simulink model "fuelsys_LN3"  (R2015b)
settings: Solver=ode45  SolverMode=SingleTasking  StartTime=0.0  StopTime=50  FixedStep=0.001  RelTol=1e-5  AbsTol=1e-6
PostLoadFcn:
  | sldemo_fuelsys_data(bdroot,'initialize_data','orig','float');
model workspace (MAT data in the model file):
  PressEst = [0.806253176324 0.553142316929 0.37151500209 0.277667903103 0.220198954207 0.181288665766 0.153200000489 0.115431020872 0.0913067476324 0.0746519188607 0.0625231108324 0.0533383634277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]
  PressVect = [0.05 0.1 0.15 0.2 0.25 0.3 0.35 0.4 0.45 0.5 0.55 0.6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]
  PumpCon = [-0.0556348 -0.0022828 0.0256932 0.0435188 0.0562692 0.0661194857143 0.0741572 0.08697 0.0972452 0.106070342857 0.1139892 0.121303866667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]
  RampRateKiX = [100 200 300 400 500 600]
  RampRateKiY = [0 0.2 0.4 0.6 0.8 1]
  RampRateKiZ = [0.012 0.024 0.036 0.048 0.06 0.072 0.024 0.048 0.072 0.096 0.12 0.144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]
  SpeedEst = [471.837839721 550.80940091 777.559313277 1080.9243499 1418.36795322 1769.7468768 2125.37309264 2480.20345067 2831.37796793 3177.14006959 3516.32917143 4064.90417867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]
  SpeedVect = [50 75 100 125 150 175 200 250 300 350 400 450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]
  ThrotEst = [0 0 0 0 0 0 0 0 0 0 0 0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]
  ThrotVect = [0 3 6 9 12 15 18 21 24 27 30 35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]
  hys = 25
  max_ego = 1.2
  max_press = 0.95
  max_speed = 628
  max_throt = 90
  min_press = 0.05
  min_speed = 50
  min_throt = 3
  st_range = 0.0001
  zero_thresh = 250
undefined symbols (not defined in the file or in its folder): DiscIntNeverNeededParam, sld_FuelModes, sldvsubsys
libraries: simulink x7, simulink_extras x2

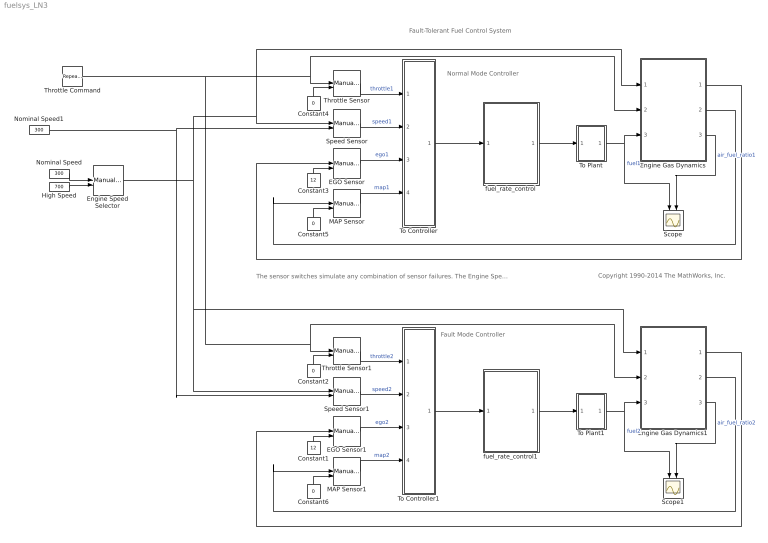
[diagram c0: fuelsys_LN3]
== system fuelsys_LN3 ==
  note: Normal Mode Controller
  note: Fault-Tolerant Fuel Control System
  note: Copyright 1990-2014 The MathWorks, Inc.
  note: The sensor switches simulate any combination of sensor failures. The Engine Speed Selector switch simulates different engine speeds (rad/sec).
  note: Fault Mode Controller
  Constant1 : Constant  Value=12
  Constant{2,4..6} (4 alike) : Constant  Value=0
  Constant3 : Constant  Value=12
  EGO Sensor : ManualSwitch
  EGO Sensor1 : ManualSwitch
  Engine Speed Selector : ManualSwitch
  Engine Gas Dynamics : Subsystem
  Engine Gas Dynamics1 : Subsystem
  High Speed : Constant  Value=700
  MAP Sensor : ManualSwitch
  MAP Sensor1 : ManualSwitch
  Nominal Speed : Constant  Value=300
  Nominal Speed1 : Constant  Value=300
  Scope : Scope  NumInputPorts=2
  Scope1 : Scope  NumInputPorts=2
  Speed Sensor : ManualSwitch  CurrentSetting=0
  Speed Sensor1 : ManualSwitch  CurrentSetting=0
  Throttle Command : simulink/Sources/Repeating Sequence  rep_seq_t=[0 2 4]  rep_seq_y=[10 20 10]
  Throttle Sensor : ManualSwitch
  Throttle Sensor1 : ManualSwitch
  To Controller : Subsystem
  To Controller1 : Subsystem
  To Plant : Subsystem
  To Plant1 : Subsystem
  fuel_rate_control : Subsystem  Tag=FuelRateControl  TreatAsAtomicUnit=on
  fuel_rate_control1 : Subsystem  Tag=FuelRateControl  TreatAsAtomicUnit=on
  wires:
  Engine Gas Dynamics/3(air/fuel ratio) -> Scope/2  "air_fuel_ratio1"
  fuel_rate_control/1(fuel_rate) -> To Plant/1(In1)
  Engine Gas Dynamics/1(o2_out) -> EGO Sensor/1
  Constant5/1 -> MAP Sensor/2
  Constant3/1 -> EGO Sensor/2
  Constant4/1 -> Throttle Sensor/2
  Engine Gas Dynamics/2(MAP) -> MAP Sensor/1
  High Speed/1 -> Engine Speed Selector/2
  Nominal Speed/1 -> Engine Speed Selector/1
  EGO Sensor/1 -> To Controller/3(ego)  "ego1"
  MAP Sensor/1 -> To Controller/4(map)  "map1"
  Throttle Sensor/1 -> To Controller/1(throttle)  "throttle1"
  Speed Sensor/1 -> To Controller/2(speed)  "speed1"
  To Plant/1(Out1) -> Scope/1, Engine Gas Dynamics/3(fuel)  "fuel1"
  To Controller/1(sensors) -> fuel_rate_control/1(sensors)
  Engine Gas Dynamics1/3(air/fuel ratio) -> Scope1/2  "air_fuel_ratio2"
  Engine Speed Selector/1 -> Engine Gas Dynamics/1(engine speed), Speed Sensor/1, Engine Gas Dynamics1/1(engine speed), Speed Sensor1/1
  fuel_rate_control1/1(fuel_rate) -> To Plant1/1(In1)
  Engine Gas Dynamics1/1(o2_out) -> EGO Sensor1/1
  Constant6/1 -> MAP Sensor1/2
  Constant1/1 -> EGO Sensor1/2
  Throttle Command/1 -> Engine Gas Dynamics/2(throttle angle), Throttle Sensor/1, Engine Gas Dynamics1/2(throttle angle), Throttle Sensor1/1
  Constant2/1 -> Throttle Sensor1/2
  Engine Gas Dynamics1/2(MAP) -> MAP Sensor1/1
  EGO Sensor1/1 -> To Controller1/3(ego)  "ego2"
  MAP Sensor1/1 -> To Controller1/4(map)  "map2"
  Throttle Sensor1/1 -> To Controller1/1(throttle)  "throttle2"
  Speed Sensor1/1 -> To Controller1/2(speed)  "speed2"
  To Plant1/1(Out1) -> Scope1/1, Engine Gas Dynamics1/3(fuel)  "fuel2"
  To Controller1/1(sensors) -> fuel_rate_control1/1(sensors)
  Nominal Speed1/1 -> Speed Sensor1/2, Speed Sensor/2

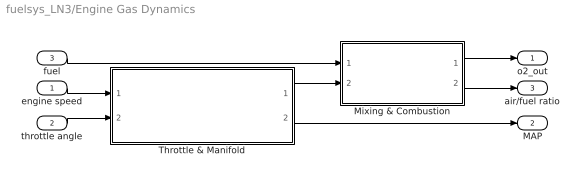
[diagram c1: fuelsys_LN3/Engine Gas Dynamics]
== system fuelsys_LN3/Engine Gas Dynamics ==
  engine speed : Inport
  throttle angle : Inport  Port=2
  fuel : Inport  Port=3
  Mixing & Combustion : Subsystem
  Throttle & Manifold : Subsystem
  o2_out : Outport
  MAP : Outport  Port=2
  air/fuel ratio : Outport  Port=3
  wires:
  Throttle & Manifold/1(Mass Airflow Rate) -> Mixing & Combustion/2(air flow)
  fuel/1 -> Mixing & Combustion/1(fuel rate)
  engine speed/1 -> Throttle & Manifold/1("Engine Speed, N")
  throttle angle/1 -> Throttle & Manifold/2(Throttle Ang.)
  Mixing & Combustion/2(air/fuel ratio) -> air/fuel ratio/1
  Throttle & Manifold/2(MAP (bar)) -> MAP/1
  Mixing & Combustion/1(o2_out) -> o2_out/1

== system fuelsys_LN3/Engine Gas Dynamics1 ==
  engine speed : Inport
  throttle angle : Inport  Port=2
  fuel : Inport  Port=3
  Mixing & Combustion : Subsystem
  Throttle & Manifold : Subsystem
  o2_out : Outport
  MAP : Outport  Port=2
  air/fuel ratio : Outport  Port=3
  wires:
  Throttle & Manifold/1(Mass Airflow Rate) -> Mixing & Combustion/2(air flow)
  fuel/1 -> Mixing & Combustion/1(fuel rate)
  engine speed/1 -> Throttle & Manifold/1("Engine Speed, N")
  throttle angle/1 -> Throttle & Manifold/2(Throttle Ang.)
  Mixing & Combustion/2(air/fuel ratio) -> air/fuel ratio/1
  Throttle & Manifold/2(MAP (bar)) -> MAP/1
  Mixing & Combustion/1(o2_out) -> o2_out/1

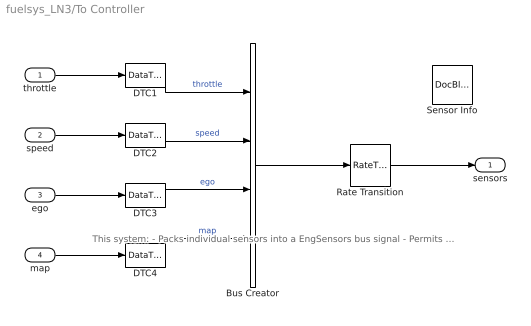
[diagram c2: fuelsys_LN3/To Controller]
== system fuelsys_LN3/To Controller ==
  note: This system: - Packs individual sensors into a EngSensors bus signal - Permits bus elements data types to change - Converts signals from continuous to discrete time
  throttle : Inport
  speed : Inport  Port=2
  ego : Inport  Port=3
  map : Inport  Port=4
  Bus Creator : BusCreator  Inputs=4  OutDataTypeStr=Bus: EngSensors
  DTC{1..4} (4 alike) : DataTypeConversion  SampleTime=[0 1]
  Rate Transition : RateTransition  OutPortSampleTime=0.01
  Sensor Info : simulink/Model-Wide Utilities/DocBlock  DocumentType=Text
  sensors : Outport
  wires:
  throttle/1 -> DTC1/1
  DTC1/1 -> Bus Creator/1  "throttle"
  speed/1 -> DTC2/1
  DTC2/1 -> Bus Creator/2  "speed"
  ego/1 -> DTC3/1
  DTC3/1 -> Bus Creator/3  "ego"
  map/1 -> DTC4/1
  DTC4/1 -> Bus Creator/4  "map"
  Bus Creator/1 -> Rate Transition/1
  Rate Transition/1 -> sensors/1

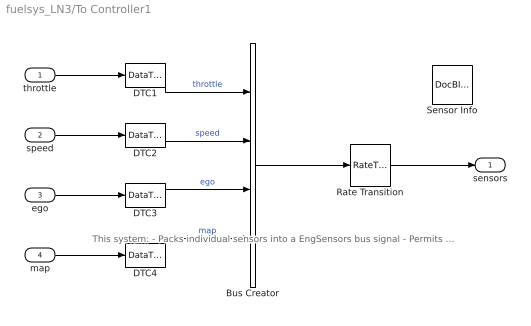
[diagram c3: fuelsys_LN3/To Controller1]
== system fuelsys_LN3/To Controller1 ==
  note: This system: - Packs individual sensors into a EngSensors bus signal - Permits bus elements data types to change - Converts signals from continuous to discrete time
  throttle : Inport
  speed : Inport  Port=2
  ego : Inport  Port=3
  map : Inport  Port=4
  Bus Creator : BusCreator  Inputs=4  OutDataTypeStr=Bus: EngSensors
  DTC{1..4} (4 alike) : DataTypeConversion  SampleTime=[0 1]
  Rate Transition : RateTransition  OutPortSampleTime=0.01
  Sensor Info : simulink/Model-Wide Utilities/DocBlock  DocumentType=Text
  sensors : Outport
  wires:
  throttle/1 -> DTC1/1
  DTC1/1 -> Bus Creator/1  "throttle"
  speed/1 -> DTC2/1
  DTC2/1 -> Bus Creator/2  "speed"
  ego/1 -> DTC3/1
  DTC3/1 -> Bus Creator/3  "ego"
  map/1 -> DTC4/1
  DTC4/1 -> Bus Creator/4  "map"
  Bus Creator/1 -> Rate Transition/1
  Rate Transition/1 -> sensors/1

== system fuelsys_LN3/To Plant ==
  note: This system: - Permits upstream signal data type to change - Converts signals from discrete to continuous time
  In1 : Inport
  DTC5 : DataTypeConversion
  Rate Transition1 : RateTransition  Integrity=off  X0=1.6  OutPortSampleTime=0
  Out1 : Outport
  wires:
  DTC5/1 -> Rate Transition1/1
  In1/1 -> DTC5/1
  Rate Transition1/1 -> Out1/1

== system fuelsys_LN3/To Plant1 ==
  note: This system: - Permits upstream signal data type to change - Converts signals from discrete to continuous time
  In1 : Inport
  DTC5 : DataTypeConversion
  Rate Transition1 : RateTransition  Integrity=off  X0=1.6  OutPortSampleTime=0
  Out1 : Outport
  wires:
  DTC5/1 -> Rate Transition1/1
  In1/1 -> DTC5/1
  Rate Transition1/1 -> Out1/1

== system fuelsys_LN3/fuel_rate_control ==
  note: Fuel Rate Control Subsystem
  sensors : Inport  OutDataTypeStr=Bus: EngSensors
  Bus Selector1 : BusSelector  OutputSignals=speed
  airflow_calc : Subsystem
  control_logic : Stateflow chart  Description=Stateflow diagram to determine control system operating mode  TreatAsAtomicUnit=on
  fuel_calc : Subsystem
  validate_sample_time : Subsystem  Tag=VerificationSubsystem  DisableCoverage=on  LoadFcn=sldvsubsys('check')  TreatAsAtomicUnit=on  SimViewingDevice=on
  fuel_rate : Outport
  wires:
  fuel_calc/1(fuel_rate) -> fuel_rate/1
  airflow_calc/1(est_airflow) -> fuel_calc/1(est_airflow)
  sensors/1 -> control_logic/1(es_i), Bus Selector1/1
  control_logic/3(fuel_mode) -> airflow_calc/3(fuel_mode), fuel_calc/3(fuel_mode)
  control_logic/1(es_o) -> airflow_calc/1(sensors)
  control_logic/2(" O2_normal") -> airflow_calc/2(O2_normal)
  airflow_calc/2(fb_correction) -> fuel_calc/2(fb_correction)
  Bus Selector1/1 -> validate_sample_time/1(In1)  "<speed>"

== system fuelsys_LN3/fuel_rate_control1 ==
  note: Fuel Rate Control Subsystem
  sensors : Inport  OutDataTypeStr=Bus: EngSensors
  Bus Selector1 : BusSelector  OutputSignals=speed
  airflow_calc : Subsystem
  control_logic : Stateflow chart  Description=Stateflow diagram to determine control system operating mode  TreatAsAtomicUnit=on
  fuel_calc : Subsystem
  validate_sample_time : Subsystem  Tag=VerificationSubsystem  DisableCoverage=on  LoadFcn=sldvsubsys('check')  TreatAsAtomicUnit=on  SimViewingDevice=on
  fuel_rate : Outport
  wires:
  fuel_calc/1(fuel_rate) -> fuel_rate/1
  airflow_calc/1(est_airflow) -> fuel_calc/1(est_airflow)
  sensors/1 -> control_logic/1(es_i), Bus Selector1/1
  control_logic/3(fuel_mode) -> airflow_calc/3(fuel_mode), fuel_calc/3(fuel_mode)
  control_logic/1(es_o) -> airflow_calc/1(sensors)
  control_logic/2(" O2_normal") -> airflow_calc/2(O2_normal)
  airflow_calc/2(fb_correction) -> fuel_calc/2(fb_correction)
  Bus Selector1/1 -> validate_sample_time/1(In1)  "<speed>"

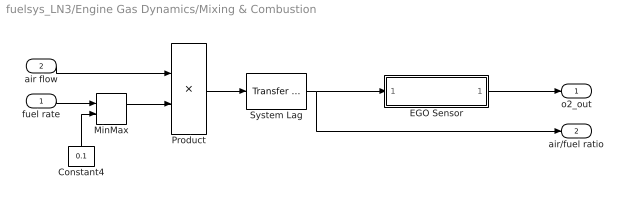
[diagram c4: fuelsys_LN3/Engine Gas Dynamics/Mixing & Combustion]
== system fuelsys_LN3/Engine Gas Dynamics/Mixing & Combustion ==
  fuel rate : Inport
  air flow : Inport  Port=2
  Constant4 : Constant  Value=0.1
  EGO Sensor : MATLAB Function  TreatAsAtomicUnit=on
  MinMax : MinMax  Function=max  Inputs=2
  Product : Product  Inputs=*/
  System Lag : simulink_extras/Additional Linear/Transfer Fcn (with initial outputs)  N=3  D=[1 3]  Y0=1/14.6  U0=1/14.6
  o2_out : Outport
  air/fuel ratio : Outport  Port=2
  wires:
  Constant4/1 -> MinMax/2
  fuel rate/1 -> MinMax/1
  MinMax/1 -> Product/2
  Product/1 -> System Lag/1
  System Lag/1 -> air/fuel ratio/1, EGO Sensor/1(u)
  EGO Sensor/1(y) -> o2_out/1
  air flow/1 -> Product/1

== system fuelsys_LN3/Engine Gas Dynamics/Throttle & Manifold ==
  note: Air-Fuel Intake Dynamics
  "Engine Speed, N" : Inport
  Throttle Ang. : Inport  Port=2
  "Atmospheric Pressure, Pa (bar)" : Constant  Value=1.0
  Intake Manifold : Subsystem
  Limit to Positive : Saturate  UpperLimit=inf  LowerLimit=0
  Throttle : Subsystem
  Mass Airflow Rate : Outport
  MAP (bar) : Outport  Port=2
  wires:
  Limit to Positive/1 -> Throttle/1("Throttle Angle, theta (deg)")
  Throttle Ang./1 -> Limit to Positive/1
  Throttle/1("Throttle Flow, mdot (g/s)") -> Intake Manifold/1(mdot Input (g/s))
  "Engine Speed, N"/1 -> Intake Manifold/2(N (rad/sec))
  Intake Manifold/1(mdot to Cylinder (g/s)) -> Mass Airflow Rate/1
  "Atmospheric Pressure, Pa (bar)"/1 -> Throttle/3("Atmospheric Pressure, Pa (bar) ")
  Intake Manifold/2("Manifold Pressure, Pm (bar)") -> Throttle/2("Manifold Pressure, Pm (bar)"), MAP (bar)/1

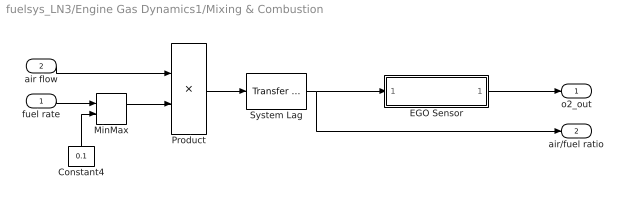
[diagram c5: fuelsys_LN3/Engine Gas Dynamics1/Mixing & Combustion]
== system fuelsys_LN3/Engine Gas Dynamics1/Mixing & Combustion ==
  fuel rate : Inport
  air flow : Inport  Port=2
  Constant4 : Constant  Value=0.1
  EGO Sensor : MATLAB Function  TreatAsAtomicUnit=on
  MinMax : MinMax  Function=max  Inputs=2
  Product : Product  Inputs=*/
  System Lag : simulink_extras/Additional Linear/Transfer Fcn (with initial outputs)  N=3  D=[1 3]  Y0=1/14.6  U0=1/14.6
  o2_out : Outport
  air/fuel ratio : Outport  Port=2
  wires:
  Constant4/1 -> MinMax/2
  fuel rate/1 -> MinMax/1
  MinMax/1 -> Product/2
  Product/1 -> System Lag/1
  System Lag/1 -> air/fuel ratio/1, EGO Sensor/1(u)
  EGO Sensor/1(y) -> o2_out/1
  air flow/1 -> Product/1

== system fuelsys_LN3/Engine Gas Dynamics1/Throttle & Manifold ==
  note: Air-Fuel Intake Dynamics
  "Engine Speed, N" : Inport
  Throttle Ang. : Inport  Port=2
  "Atmospheric Pressure, Pa (bar)" : Constant  Value=1.0
  Intake Manifold : Subsystem
  Limit to Positive : Saturate  UpperLimit=inf  LowerLimit=0
  Throttle : Subsystem
  Mass Airflow Rate : Outport
  MAP (bar) : Outport  Port=2
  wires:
  Limit to Positive/1 -> Throttle/1("Throttle Angle, theta (deg)")
  Throttle Ang./1 -> Limit to Positive/1
  Throttle/1("Throttle Flow, mdot (g/s)") -> Intake Manifold/1(mdot Input (g/s))
  "Engine Speed, N"/1 -> Intake Manifold/2(N (rad/sec))
  Intake Manifold/1(mdot to Cylinder (g/s)) -> Mass Airflow Rate/1
  "Atmospheric Pressure, Pa (bar)"/1 -> Throttle/3("Atmospheric Pressure, Pa (bar) ")
  Intake Manifold/2("Manifold Pressure, Pm (bar)") -> Throttle/2("Manifold Pressure, Pm (bar)"), MAP (bar)/1

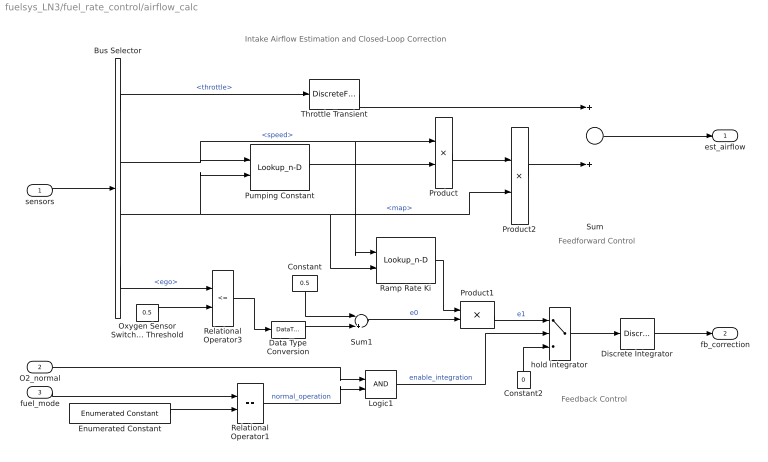
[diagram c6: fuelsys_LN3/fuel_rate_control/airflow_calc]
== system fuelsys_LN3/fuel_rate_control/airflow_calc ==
  note: Intake Airflow Estimation and Closed-Loop Correction
  note: Feedback Control
  note: Feedforward Control
  sensors : Inport
  O2_normal : Inport  Port=2
  fuel_mode : Inport  Port=3
  Bus Selector : BusSelector  OutputSignals=throttle,speed,map,ego
  Constant : Constant  Value=0.5  OutDataTypeStr=s16En7
  Constant2 : Constant  Value=0  OutDataTypeStr=uint8
  Data Type Conversion : DataTypeConversion  OutDataTypeStr=s16En7  RndMeth=Simplest
  Discrete Integrator : DiscreteIntegrator  InitialConditionSetting=State (most efficient)  SampleTime=-1  OutDataTypeStr=s16En15  RndMeth=Simplest  ICPrevOutput=DiscIntNeverNeededParam  ICPrevScaledInput=DiscIntNeverNeededParam
  Enumerated Constant : simulink/Sources/Enumerated Constant  OutDataTypeStr=Enum: sld_FuelModes  Value=sld_FuelModes.LOW  SampleTime=.01
  Logic1 : Logic  IconShape=distinctive  AllPortsSameDT=off  OutDataTypeStr=boolean
  Oxygen Sensor Switching Threshold : Constant  Value=0.5  OutDataTypeStr=s16En7
  Product : Product  OutDataTypeStr=s16En7  RndMeth=Simplest
  Product1 : Product  OutDataTypeStr=s16En15  RndMeth=Simplest
  Product2 : Product  OutDataTypeStr=s16En7  RndMeth=Simplest
  Pumping Constant : Lookup_n-D  BreakpointsForDimension1=SpeedVect  BreakpointsForDimension2=PressVect  IndexSearchMethod=Linear search  Table=PumpCon  ExtrapMethod=Clip  UseLastTableValue=on  OutDataTypeStr=s16En15  RndMeth=Simplest
  Ramp Rate Ki : Lookup_n-D  BreakpointsForDimension1=RampRateKiX  BreakpointsForDimension2=RampRateKiY  IndexSearchMethod=Linear search  Table=RampRateKiZ  ExtrapMethod=Clip  UseLastTableValue=on  OutDataTypeStr=s16En15  RndMeth=Simplest
  Relational Operator1 : RelationalOperator  Operator===  OutDataTypeStr=boolean
  Relational Operator3 : RelationalOperator  Operator=<=  OutDataTypeStr=boolean
  Sum : Sum  Inputs=2  OutDataTypeStr=s16En7  RndMeth=Simplest
  Sum1 : Sum  Inputs=-+  OutDataTypeStr=s16En15  RndMeth=Simplest
  Throttle Transient : DiscreteFilter  Numerator=[.01 -.01]  Denominator=[1 -.8]  a0EqualsOne=on  OutDataTypeStr=s16En7  RndMeth=Simplest
  hold integrator : Switch  Criteria=u2 ~= 0  Threshold=1  OutDataTypeStr=s16En15  RndMeth=Simplest
  est_airflow : Outport
  fb_correction : Outport  Port=2
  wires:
  Discrete Integrator/1 -> fb_correction/1
  sensors/1 -> Bus Selector/1
  Pumping Constant/1 -> Product/2
  Bus Selector/2 -> Product/1, Ramp Rate Ki/1, Pumping Constant/1  "<speed>"
  Throttle Transient/1 -> Sum/1
  Sum/1 -> est_airflow/1
  Bus Selector/1 -> Throttle Transient/1  "<throttle>"
  Relational Operator1/1 -> Logic1/2  "normal_operation"
  Oxygen Sensor Switching Threshold/1 -> Relational Operator3/2
  Constant/1 -> Sum1/1
  Ramp Rate Ki/1 -> Product1/1
  Constant2/1 -> hold integrator/3
  Product1/1 -> hold integrator/1  "e1"
  hold integrator/1 -> Discrete Integrator/1
  Logic1/1 -> hold integrator/2  "enable_integration"
  Sum1/1 -> Product1/2  "e0"
  Relational Operator3/1 -> Data Type Conversion/1
  Data Type Conversion/1 -> Sum1/2
  Bus Selector/3 -> Product2/2, Ramp Rate Ki/2, Pumping Constant/2  "<map>"
  Bus Selector/4 -> Relational Operator3/1  "<ego>"
  Product/1 -> Product2/1
  Product2/1 -> Sum/2
  O2_normal/1 -> Logic1/1
  Enumerated Constant/1 -> Relational Operator1/2
  fuel_mode/1 -> Relational Operator1/1

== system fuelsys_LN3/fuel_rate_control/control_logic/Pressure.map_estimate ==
  note: MAP Estimation
  speed : Inport  OutDataTypeStr=s16En3
  throttle : Inport  Port=2  OutDataTypeStr=s16En3
  f : TriggerPort  TriggerType=function-call
  Pressure Estimation : Lookup_n-D  BreakpointsForDimension1=SpeedVect  BreakpointsForDimension2=ThrotVect  IndexSearchMethod=Linear search  Table=PressEst  ExtrapMethod=Clip  UseLastTableValue=on  OutDataTypeStr=u8En7  RndMeth=Simplest
  map : Outport
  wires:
  speed/1 -> Pressure Estimation/1
  throttle/1 -> Pressure Estimation/2
  Pressure Estimation/1 -> map/1

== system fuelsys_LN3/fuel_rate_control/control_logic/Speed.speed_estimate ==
  note: Speed Estimation
  throttle : Inport  OutDataTypeStr=s16En3
  map : Inport  Port=2  OutDataTypeStr=u8En7
  f : TriggerPort  TriggerType=function-call
  Saturation : Saturate  UpperLimit=max_speed  LowerLimit=0  OutDataTypeStr=s16En3
  Speed Estimation : Lookup_n-D  BreakpointsForDimension1=ThrotVect  BreakpointsForDimension2=PressVect  IndexSearchMethod=Linear search  Table=SpeedEst  ExtrapMethod=Clip  UseLastTableValue=on  OutDataTypeStr=s16En3  RndMeth=Simplest
  speed : Outport
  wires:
  Speed Estimation/1 -> Saturation/1
  throttle/1 -> Speed Estimation/1
  map/1 -> Speed Estimation/2
  Saturation/1 -> speed/1

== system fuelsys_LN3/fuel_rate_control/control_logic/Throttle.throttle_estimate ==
  note: Throttle Estimation
  speed : Inport  OutDataTypeStr=s16En3
  map : Inport  Port=2  OutDataTypeStr=u8En7
  f : TriggerPort  TriggerType=function-call
  Throttle Estimation : Lookup_n-D  BreakpointsForDimension1=SpeedVect  BreakpointsForDimension2=PressVect  IndexSearchMethod=Linear search  Table=ThrotEst  ExtrapMethod=Clip  UseLastTableValue=on  OutDataTypeStr=s16En7  RndMeth=Simplest
  throttle : Outport
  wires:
  speed/1 -> Throttle Estimation/1
  map/1 -> Throttle Estimation/2
  Throttle Estimation/1 -> throttle/1

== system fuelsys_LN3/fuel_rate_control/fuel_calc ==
  note: Fuel Rate Calculation
  est_airflow : Inport
  fb_correction : Inport  Port=2
  fuel_mode : Inport  Port=3
  feedforward_fuel_rate : Subsystem
  switchable_compensation : Subsystem
  fuel_rate : Outport
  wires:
  est_airflow/1 -> feedforward_fuel_rate/1(est_airflow)
  fuel_mode/1 -> feedforward_fuel_rate/2(fuel_mode), switchable_compensation/2(fuel_mode)
  switchable_compensation/1(fuel_rate) -> fuel_rate/1
  fb_correction/1 -> switchable_compensation/3(fb_correction)
  feedforward_fuel_rate/1(ff_fuel_rate) -> switchable_compensation/1(ff_fuel_rate)

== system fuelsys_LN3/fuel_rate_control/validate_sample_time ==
  note: The contents of this subsystem are excluded from the code Simulink Coder generates. To work correctly this system must continue to * Contain no output ports * Enable its 'Treat as Atomic Unit' parameter * Specify its 'Mask type' parameter as "VerificationSubsystem"
  note: Verify sample time: aspects of the design assume a 0.01 second sample time.
  In1 : Inport
  Actual Sample Time : Probe  ProbeWidth=off  ProbeComplexSignal=off  ProbeSampleTimeDataType=Same as input
  CheckRange : simulink/Model Verification/Check  Static Range  Description=-st_range < u < st_range  max=st_range  max_included=off  min=-st_range  min_included=off  enabled=on  stopWhenAssertionFail=on  export=off  icon=graphic
  Data Type Conversion : DataTypeConversion  OutDataTypeStr=s16En15
  Demux : Demux  Outputs=2
  Expected Sample Time : Constant  Value=0.01  OutDataTypeStr=s16En15
  Sum : Sum  Inputs=|+-
  Terminator : Terminator
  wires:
  Actual Sample Time/1 -> Demux/1
  In1/1 -> Data Type Conversion/1
  Demux/2 -> Terminator/1
  Demux/1 -> Sum/1
  Expected Sample Time/1 -> Sum/2
  Sum/1 -> CheckRange/1
  Data Type Conversion/1 -> Actual Sample Time/1

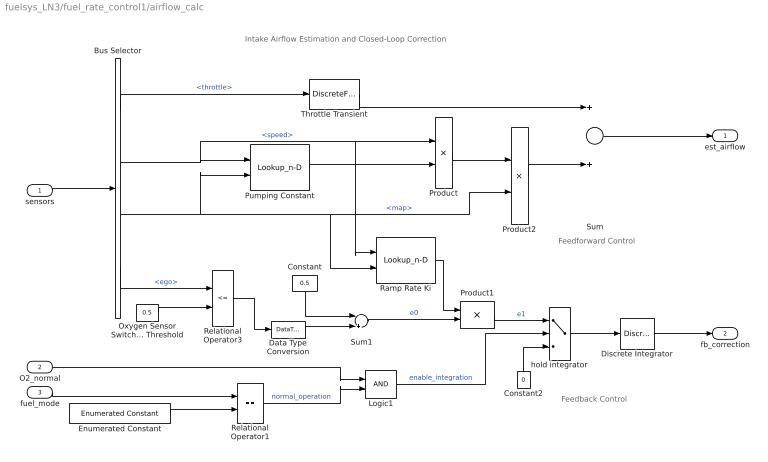
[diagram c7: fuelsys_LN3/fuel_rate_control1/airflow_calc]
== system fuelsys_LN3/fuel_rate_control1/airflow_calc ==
  note: Intake Airflow Estimation and Closed-Loop Correction
  note: Feedback Control
  note: Feedforward Control
  sensors : Inport
  O2_normal : Inport  Port=2
  fuel_mode : Inport  Port=3
  Bus Selector : BusSelector  OutputSignals=throttle,speed,map,ego
  Constant : Constant  Value=0.5  OutDataTypeStr=s16En7
  Constant2 : Constant  Value=0  OutDataTypeStr=uint8
  Data Type Conversion : DataTypeConversion  OutDataTypeStr=s16En7  RndMeth=Simplest
  Discrete Integrator : DiscreteIntegrator  InitialConditionSetting=State (most efficient)  SampleTime=-1  OutDataTypeStr=s16En15  RndMeth=Simplest  ICPrevOutput=DiscIntNeverNeededParam  ICPrevScaledInput=DiscIntNeverNeededParam
  Enumerated Constant : simulink/Sources/Enumerated Constant  OutDataTypeStr=Enum: sld_FuelModes  Value=sld_FuelModes.LOW  SampleTime=.01
  Logic1 : Logic  IconShape=distinctive  AllPortsSameDT=off  OutDataTypeStr=boolean
  Oxygen Sensor Switching Threshold : Constant  Value=0.5  OutDataTypeStr=s16En7
  Product : Product  OutDataTypeStr=s16En7  RndMeth=Simplest
  Product1 : Product  OutDataTypeStr=s16En15  RndMeth=Simplest
  Product2 : Product  OutDataTypeStr=s16En7  RndMeth=Simplest
  Pumping Constant : Lookup_n-D  BreakpointsForDimension1=SpeedVect  BreakpointsForDimension2=PressVect  IndexSearchMethod=Linear search  Table=PumpCon  ExtrapMethod=Clip  UseLastTableValue=on  OutDataTypeStr=s16En15  RndMeth=Simplest
  Ramp Rate Ki : Lookup_n-D  BreakpointsForDimension1=RampRateKiX  BreakpointsForDimension2=RampRateKiY  IndexSearchMethod=Linear search  Table=RampRateKiZ  ExtrapMethod=Clip  UseLastTableValue=on  OutDataTypeStr=s16En15  RndMeth=Simplest
  Relational Operator1 : RelationalOperator  Operator===  OutDataTypeStr=boolean
  Relational Operator3 : RelationalOperator  Operator=<=  OutDataTypeStr=boolean
  Sum : Sum  Inputs=2  OutDataTypeStr=s16En7  RndMeth=Simplest
  Sum1 : Sum  Inputs=-+  OutDataTypeStr=s16En15  RndMeth=Simplest
  Throttle Transient : DiscreteFilter  Numerator=[.01 -.01]  Denominator=[1 -.8]  a0EqualsOne=on  OutDataTypeStr=s16En7  RndMeth=Simplest
  hold integrator : Switch  Criteria=u2 ~= 0  Threshold=1  OutDataTypeStr=s16En15  RndMeth=Simplest
  est_airflow : Outport
  fb_correction : Outport  Port=2
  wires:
  Discrete Integrator/1 -> fb_correction/1
  sensors/1 -> Bus Selector/1
  Pumping Constant/1 -> Product/2
  Bus Selector/2 -> Product/1, Ramp Rate Ki/1, Pumping Constant/1  "<speed>"
  Throttle Transient/1 -> Sum/1
  Sum/1 -> est_airflow/1
  Bus Selector/1 -> Throttle Transient/1  "<throttle>"
  Relational Operator1/1 -> Logic1/2  "normal_operation"
  Oxygen Sensor Switching Threshold/1 -> Relational Operator3/2
  Constant/1 -> Sum1/1
  Ramp Rate Ki/1 -> Product1/1
  Constant2/1 -> hold integrator/3
  Product1/1 -> hold integrator/1  "e1"
  hold integrator/1 -> Discrete Integrator/1
  Logic1/1 -> hold integrator/2  "enable_integration"
  Sum1/1 -> Product1/2  "e0"
  Relational Operator3/1 -> Data Type Conversion/1
  Data Type Conversion/1 -> Sum1/2
  Bus Selector/3 -> Product2/2, Ramp Rate Ki/2, Pumping Constant/2  "<map>"
  Bus Selector/4 -> Relational Operator3/1  "<ego>"
  Product/1 -> Product2/1
  Product2/1 -> Sum/2
  O2_normal/1 -> Logic1/1
  Enumerated Constant/1 -> Relational Operator1/2
  fuel_mode/1 -> Relational Operator1/1

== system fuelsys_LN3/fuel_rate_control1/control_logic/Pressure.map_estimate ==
  note: MAP Estimation
  speed : Inport  OutDataTypeStr=s16En3
  throttle : Inport  Port=2  OutDataTypeStr=s16En3
  f : TriggerPort  TriggerType=function-call
  Pressure Estimation : Lookup_n-D  BreakpointsForDimension1=SpeedVect  BreakpointsForDimension2=ThrotVect  IndexSearchMethod=Linear search  Table=PressEst  ExtrapMethod=Clip  UseLastTableValue=on  OutDataTypeStr=u8En7  RndMeth=Simplest
  map : Outport
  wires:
  speed/1 -> Pressure Estimation/1
  throttle/1 -> Pressure Estimation/2
  Pressure Estimation/1 -> map/1

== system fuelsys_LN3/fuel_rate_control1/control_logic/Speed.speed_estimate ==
  note: Speed Estimation
  throttle : Inport  OutDataTypeStr=s16En3
  map : Inport  Port=2  OutDataTypeStr=u8En7
  f : TriggerPort  TriggerType=function-call
  Saturation : Saturate  UpperLimit=max_speed  LowerLimit=0  OutDataTypeStr=s16En3
  Speed Estimation : Lookup_n-D  BreakpointsForDimension1=ThrotVect  BreakpointsForDimension2=PressVect  IndexSearchMethod=Linear search  Table=SpeedEst  ExtrapMethod=Clip  UseLastTableValue=on  OutDataTypeStr=s16En3  RndMeth=Simplest
  speed : Outport
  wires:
  Speed Estimation/1 -> Saturation/1
  throttle/1 -> Speed Estimation/1
  map/1 -> Speed Estimation/2
  Saturation/1 -> speed/1

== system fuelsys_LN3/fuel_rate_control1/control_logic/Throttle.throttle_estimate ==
  note: Throttle Estimation
  speed : Inport  OutDataTypeStr=s16En3
  map : Inport  Port=2  OutDataTypeStr=u8En7
  f : TriggerPort  TriggerType=function-call
  Throttle Estimation : Lookup_n-D  BreakpointsForDimension1=SpeedVect  BreakpointsForDimension2=PressVect  IndexSearchMethod=Linear search  Table=ThrotEst  ExtrapMethod=Clip  UseLastTableValue=on  OutDataTypeStr=s16En7  RndMeth=Simplest
  throttle : Outport
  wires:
  speed/1 -> Throttle Estimation/1
  map/1 -> Throttle Estimation/2
  Throttle Estimation/1 -> throttle/1

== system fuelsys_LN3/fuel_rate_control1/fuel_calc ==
  note: Fuel Rate Calculation
  est_airflow : Inport
  fb_correction : Inport  Port=2
  fuel_mode : Inport  Port=3
  feedforward_fuel_rate : Subsystem
  switchable_compensation : Subsystem
  fuel_rate : Outport
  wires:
  est_airflow/1 -> feedforward_fuel_rate/1(est_airflow)
  fuel_mode/1 -> feedforward_fuel_rate/2(fuel_mode), switchable_compensation/2(fuel_mode)
  switchable_compensation/1(fuel_rate) -> fuel_rate/1
  fb_correction/1 -> switchable_compensation/3(fb_correction)
  feedforward_fuel_rate/1(ff_fuel_rate) -> switchable_compensation/1(ff_fuel_rate)

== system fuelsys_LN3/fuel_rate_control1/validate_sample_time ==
  note: The contents of this subsystem are excluded from the code Simulink Coder generates. To work correctly this system must continue to * Contain no output ports * Enable its 'Treat as Atomic Unit' parameter * Specify its 'Mask type' parameter as "VerificationSubsystem"
  note: Verify sample time: aspects of the design assume a 0.01 second sample time.
  In1 : Inport
  Actual Sample Time : Probe  ProbeWidth=off  ProbeComplexSignal=off  ProbeSampleTimeDataType=Same as input
  CheckRange : simulink/Model Verification/Check  Static Range  Description=-st_range < u < st_range  max=st_range  max_included=off  min=-st_range  min_included=off  enabled=on  stopWhenAssertionFail=on  export=off  icon=graphic
  Data Type Conversion : DataTypeConversion  OutDataTypeStr=s16En15
  Demux : Demux  Outputs=2
  Expected Sample Time : Constant  Value=0.01  OutDataTypeStr=s16En15
  Sum : Sum  Inputs=|+-
  Terminator : Terminator
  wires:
  Actual Sample Time/1 -> Demux/1
  In1/1 -> Data Type Conversion/1
  Demux/2 -> Terminator/1
  Demux/1 -> Sum/1
  Expected Sample Time/1 -> Sum/2
  Sum/1 -> CheckRange/1
  Data Type Conversion/1 -> Actual Sample Time/1

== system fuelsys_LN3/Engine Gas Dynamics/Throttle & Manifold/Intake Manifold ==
  note: Intake Manifold Vacuum
  mdot Input (g/s) : Inport
  N (rad/sec) : Inport  Port=2
  MATLAB Function : MATLAB Function  TreatAsAtomicUnit=on
  RT/Vm : Gain  Gain=0.41328
  Sum : Sum  Inputs=+-
  p0 = 0.589 bar : Integrator  InitialCondition=.589
  mdot to Cylinder (g/s) : Outport
  "Manifold Pressure, Pm (bar)" : Outport  Port=2
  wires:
  mdot Input (g/s)/1 -> Sum/1
  RT/Vm/1 -> p0 = 0.589 bar/1
  N (rad/sec)/1 -> MATLAB Function/2(u2)
  p0 = 0.589 bar/1 -> "Manifold Pressure, Pm (bar)"/1, MATLAB Function/1(u1)
  Sum/1 -> RT/Vm/1
  MATLAB Function/1(y) -> mdot to Cylinder (g/s)/1, Sum/2

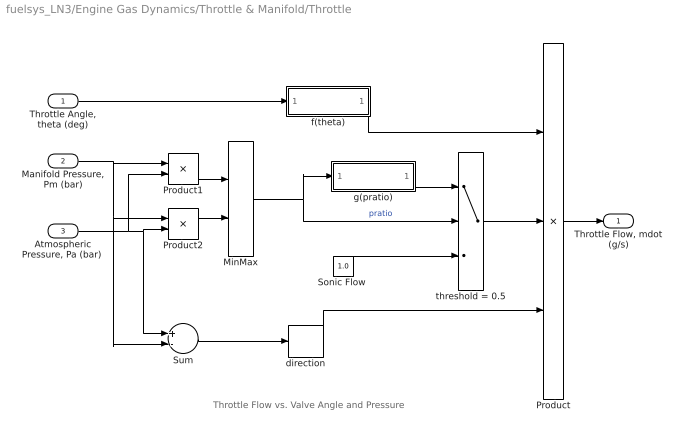
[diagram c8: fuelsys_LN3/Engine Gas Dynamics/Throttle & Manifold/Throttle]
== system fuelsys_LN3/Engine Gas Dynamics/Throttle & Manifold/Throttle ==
  note: Throttle Flow vs. Valve Angle and Pressure
  "Throttle Angle, theta (deg)" : Inport
  "Manifold Pressure, Pm (bar)" : Inport  Port=2
  "Atmospheric Pressure, Pa (bar) " : Inport  Port=3
  MinMax : MinMax  Inputs=2
  Product : Product  Inputs=3
  Product1 : Product  Inputs=*/
  Product2 : Product  Inputs=/*
  "Sonic Flow " : Constant  Value=1.0
  Sum : Sum  Inputs=+-
  direction : Signum
  f(theta) : MATLAB Function  TreatAsAtomicUnit=on
  g(pratio) : MATLAB Function  TreatAsAtomicUnit=on
  threshold = 0.5 : Switch  Threshold=0.5
  "Throttle Flow, mdot (g/s)" : Outport
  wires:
  "Manifold Pressure, Pm (bar)"/1 -> Sum/2, Product2/1, Product1/1
  Product2/1 -> MinMax/2
  Product1/1 -> MinMax/1
  "Atmospheric Pressure, Pa (bar) "/1 -> Sum/1, Product2/2, Product1/2
  g(pratio)/1(y) -> threshold = 0.5/1
  "Sonic Flow "/1 -> threshold = 0.5/3
  threshold = 0.5/1 -> Product/2
  direction/1 -> Product/3
  Sum/1 -> direction/1
  MinMax/1 -> threshold = 0.5/2, g(pratio)/1(u)  "pratio"
  "Throttle Angle, theta (deg)"/1 -> f(theta)/1(u)
  Product/1 -> "Throttle Flow, mdot (g/s)"/1
  f(theta)/1(y) -> Product/1

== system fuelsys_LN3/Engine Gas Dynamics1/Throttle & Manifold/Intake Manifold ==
  note: Intake Manifold Vacuum
  mdot Input (g/s) : Inport
  N (rad/sec) : Inport  Port=2
  MATLAB Function : MATLAB Function  TreatAsAtomicUnit=on
  RT/Vm : Gain  Gain=0.41328
  Sum : Sum  Inputs=+-
  p0 = 0.589 bar : Integrator  InitialCondition=.589
  mdot to Cylinder (g/s) : Outport
  "Manifold Pressure, Pm (bar)" : Outport  Port=2
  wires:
  mdot Input (g/s)/1 -> Sum/1
  RT/Vm/1 -> p0 = 0.589 bar/1
  N (rad/sec)/1 -> MATLAB Function/2(u2)
  p0 = 0.589 bar/1 -> "Manifold Pressure, Pm (bar)"/1, MATLAB Function/1(u1)
  Sum/1 -> RT/Vm/1
  MATLAB Function/1(y) -> mdot to Cylinder (g/s)/1, Sum/2

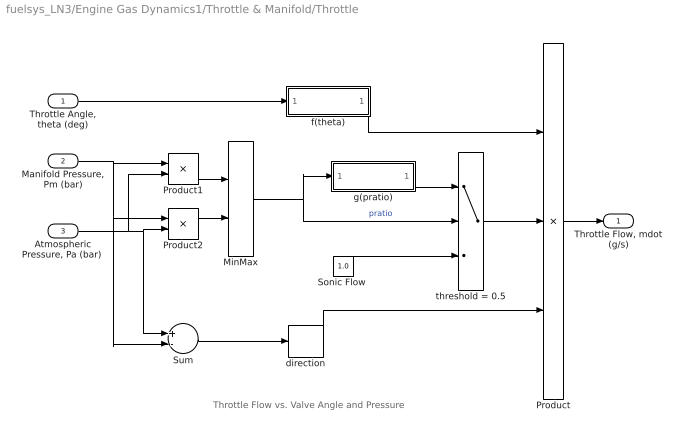
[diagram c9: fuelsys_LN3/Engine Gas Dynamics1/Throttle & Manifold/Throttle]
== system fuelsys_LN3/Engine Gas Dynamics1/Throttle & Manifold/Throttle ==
  note: Throttle Flow vs. Valve Angle and Pressure
  "Throttle Angle, theta (deg)" : Inport
  "Manifold Pressure, Pm (bar)" : Inport  Port=2
  "Atmospheric Pressure, Pa (bar) " : Inport  Port=3
  MinMax : MinMax  Inputs=2
  Product : Product  Inputs=3
  Product1 : Product  Inputs=*/
  Product2 : Product  Inputs=/*
  "Sonic Flow " : Constant  Value=1.0
  Sum : Sum  Inputs=+-
  direction : Signum
  f(theta) : MATLAB Function  TreatAsAtomicUnit=on
  g(pratio) : MATLAB Function  TreatAsAtomicUnit=on
  threshold = 0.5 : Switch  Threshold=0.5
  "Throttle Flow, mdot (g/s)" : Outport
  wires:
  "Manifold Pressure, Pm (bar)"/1 -> Sum/2, Product2/1, Product1/1
  Product2/1 -> MinMax/2
  Product1/1 -> MinMax/1
  "Atmospheric Pressure, Pa (bar) "/1 -> Sum/1, Product2/2, Product1/2
  g(pratio)/1(y) -> threshold = 0.5/1
  "Sonic Flow "/1 -> threshold = 0.5/3
  threshold = 0.5/1 -> Product/2
  direction/1 -> Product/3
  Sum/1 -> direction/1
  MinMax/1 -> threshold = 0.5/2, g(pratio)/1(u)  "pratio"
  "Throttle Angle, theta (deg)"/1 -> f(theta)/1(u)
  Product/1 -> "Throttle Flow, mdot (g/s)"/1
  f(theta)/1(y) -> Product/1

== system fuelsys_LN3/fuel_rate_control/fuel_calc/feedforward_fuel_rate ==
  note: Feedforward Fuel Rate
  est_airflow : Inport
  fuel_mode : Inport  Port=2
  Multiport Switch : MultiPortSwitch  DataPortOrder=Specify indices  DataPortIndices={sld_FuelModes.LOW, sld_FuelModes.RICH, sld_FuelModes.DISABLED}  OutDataTypeStr=s16En7  RndMeth=Simplest
  Product : Product  OutDataTypeStr=s16En7  RndMeth=Simplest
  normal : Constant  Value=1/14.6  OutDataTypeStr=s16En7
  rich : Constant  Value=1/(14.6*0.8)  OutDataTypeStr=s16En7
  shutdown : Constant  Value=0  OutDataTypeStr=s16En7
  ff_fuel_rate : Outport
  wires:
  rich/1 -> Multiport Switch/3
  fuel_mode/1 -> Multiport Switch/1
  est_airflow/1 -> Product/1
  Product/1 -> ff_fuel_rate/1
  Multiport Switch/1 -> Product/2
  normal/1 -> Multiport Switch/2
  shutdown/1 -> Multiport Switch/4

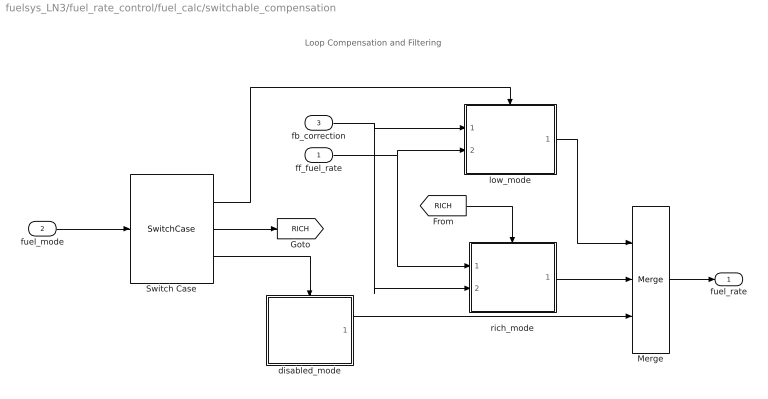
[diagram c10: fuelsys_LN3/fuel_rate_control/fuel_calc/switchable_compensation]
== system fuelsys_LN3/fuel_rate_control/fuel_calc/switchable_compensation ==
  note: Loop Compensation and Filtering
  ff_fuel_rate : Inport
  fuel_mode : Inport  Port=2
  fb_correction : Inport  Port=3
  Merge : Merge  Inputs=3
  Switch Case : SwitchCase  CaseConditions={sld_FuelModes.LOW, sld_FuelModes.RICH}
  disabled_mode : Subsystem  TreatAsAtomicUnit=on
  low_mode : Subsystem  TreatAsAtomicUnit=on
  rich_mode : Subsystem  TreatAsAtomicUnit=on
  fuel_rate : Outport
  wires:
  fuel_mode/1 -> Switch Case/1
  ff_fuel_rate/1 -> rich_mode/1(ff_fuel_rate), low_mode/2(ff_fuel_rate)
  fb_correction/1 -> rich_mode/2(fb_correction), low_mode/1(fb_correction)
  Switch Case/1 -> low_mode/Action
  Switch Case/2 -> [RICH]
  [RICH] -> rich_mode/Action
  Switch Case/3 -> disabled_mode/Action
  rich_mode/1(fuel_rate) -> Merge/2
  disabled_mode/1(fuel_rate) -> Merge/3
  low_mode/1(fuel_rate) -> Merge/1
  Merge/1 -> fuel_rate/1

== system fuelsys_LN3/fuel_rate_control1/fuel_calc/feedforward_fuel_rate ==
  note: Feedforward Fuel Rate
  est_airflow : Inport
  fuel_mode : Inport  Port=2
  Multiport Switch : MultiPortSwitch  DataPortOrder=Specify indices  DataPortIndices={sld_FuelModes.LOW, sld_FuelModes.RICH, sld_FuelModes.DISABLED}  OutDataTypeStr=s16En7  RndMeth=Simplest
  Product : Product  OutDataTypeStr=s16En7  RndMeth=Simplest
  normal : Constant  Value=1/14.6  OutDataTypeStr=s16En7
  rich : Constant  Value=1/(14.6*0.8)  OutDataTypeStr=s16En7
  shutdown : Constant  Value=0  OutDataTypeStr=s16En7
  ff_fuel_rate : Outport
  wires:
  rich/1 -> Multiport Switch/3
  fuel_mode/1 -> Multiport Switch/1
  est_airflow/1 -> Product/1
  Product/1 -> ff_fuel_rate/1
  Multiport Switch/1 -> Product/2
  normal/1 -> Multiport Switch/2
  shutdown/1 -> Multiport Switch/4

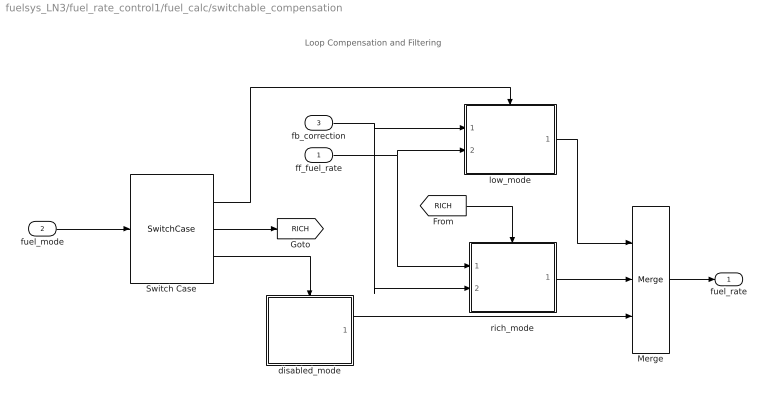
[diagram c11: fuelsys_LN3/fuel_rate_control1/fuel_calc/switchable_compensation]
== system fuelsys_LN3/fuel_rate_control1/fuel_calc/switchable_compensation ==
  note: Loop Compensation and Filtering
  ff_fuel_rate : Inport
  fuel_mode : Inport  Port=2
  fb_correction : Inport  Port=3
  Merge : Merge  Inputs=3
  Switch Case : SwitchCase  CaseConditions={sld_FuelModes.LOW, sld_FuelModes.RICH}
  disabled_mode : Subsystem  TreatAsAtomicUnit=on
  low_mode : Subsystem  TreatAsAtomicUnit=on
  rich_mode : Subsystem  TreatAsAtomicUnit=on
  fuel_rate : Outport
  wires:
  fuel_mode/1 -> Switch Case/1
  ff_fuel_rate/1 -> rich_mode/1(ff_fuel_rate), low_mode/2(ff_fuel_rate)
  fb_correction/1 -> rich_mode/2(fb_correction), low_mode/1(fb_correction)
  Switch Case/1 -> low_mode/Action
  Switch Case/2 -> [RICH]
  [RICH] -> rich_mode/Action
  Switch Case/3 -> disabled_mode/Action
  rich_mode/1(fuel_rate) -> Merge/2
  disabled_mode/1(fuel_rate) -> Merge/3
  low_mode/1(fuel_rate) -> Merge/1
  Merge/1 -> fuel_rate/1

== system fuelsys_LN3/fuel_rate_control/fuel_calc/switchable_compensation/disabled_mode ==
  note: Disabled Mode Fuel Mode
  Action Port : ActionPort  ActionType=default
  shutoff : Constant  Value=0  OutDataTypeStr=Inherit: Inherit via back propagation
  fuel_rate : Outport  InitialOutput=0
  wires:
  shutoff/1 -> fuel_rate/1

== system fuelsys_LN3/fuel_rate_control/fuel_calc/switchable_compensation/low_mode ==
  note: Low Mode Fuel Mode
  fb_correction : Inport
  ff_fuel_rate : Inport  Port=2
  Action Port : ActionPort  ActionType=case
  Discrete Filter : DiscreteFilter  Numerator=[8.7696 -8.5104]  Denominator=[1 -0.7408]  a0EqualsOne=on  RndMeth=Simplest
  Sum3 : Sum  OutDataTypeStr=s16En7  RndMeth=Simplest
  fuel_rate : Outport  InitialOutput=0
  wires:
  ff_fuel_rate/1 -> Sum3/2
  Discrete Filter/1 -> Sum3/1
  Sum3/1 -> fuel_rate/1
  fb_correction/1 -> Discrete Filter/1

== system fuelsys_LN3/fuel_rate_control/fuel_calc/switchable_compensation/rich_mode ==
  note: Rich Mode Fuel Mode
  ff_fuel_rate : Inport
  fb_correction : Inport  Port=2
  Action Port : ActionPort  ActionType=case
  Discrete Filter : DiscreteFilter  Numerator=[0 0.2592]  Denominator=[1 -0.7408]  a0EqualsOne=on  RndMeth=Simplest
  Sum2 : Sum  OutDataTypeStr=s16En7  RndMeth=Simplest
  fuel_rate : Outport  InitialOutput=0
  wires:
  fb_correction/1 -> Sum2/2
  ff_fuel_rate/1 -> Sum2/1
  Sum2/1 -> Discrete Filter/1
  Discrete Filter/1 -> fuel_rate/1

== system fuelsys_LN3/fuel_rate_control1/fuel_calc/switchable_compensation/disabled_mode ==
  note: Disabled Mode Fuel Mode
  Action Port : ActionPort  ActionType=default
  shutoff : Constant  Value=0  OutDataTypeStr=Inherit: Inherit via back propagation
  fuel_rate : Outport  InitialOutput=0
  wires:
  shutoff/1 -> fuel_rate/1

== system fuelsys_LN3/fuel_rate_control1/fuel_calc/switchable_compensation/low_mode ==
  note: Low Mode Fuel Mode
  fb_correction : Inport
  ff_fuel_rate : Inport  Port=2
  Action Port : ActionPort  ActionType=case
  Discrete Filter : DiscreteFilter  Numerator=[8.7696 -8.5104]  Denominator=[1 -0.7408]  a0EqualsOne=on  RndMeth=Simplest
  Sum3 : Sum  OutDataTypeStr=s16En7  RndMeth=Simplest
  fuel_rate : Outport  InitialOutput=0
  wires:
  ff_fuel_rate/1 -> Sum3/2
  Discrete Filter/1 -> Sum3/1
  Sum3/1 -> fuel_rate/1
  fb_correction/1 -> Discrete Filter/1

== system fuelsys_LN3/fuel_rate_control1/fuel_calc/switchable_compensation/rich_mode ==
  note: Rich Mode Fuel Mode
  ff_fuel_rate : Inport
  fb_correction : Inport  Port=2
  Action Port : ActionPort  ActionType=case
  Discrete Filter : DiscreteFilter  Numerator=[0 0.2592]  Denominator=[1 -0.7408]  a0EqualsOne=on  RndMeth=Simplest
  Sum2 : Sum  OutDataTypeStr=s16En7  RndMeth=Simplest
  fuel_rate : Outport  InitialOutput=0
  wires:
  fb_correction/1 -> Sum2/2
  ff_fuel_rate/1 -> Sum2/1
  Sum2/1 -> Discrete Filter/1
  Discrete Filter/1 -> fuel_rate/1

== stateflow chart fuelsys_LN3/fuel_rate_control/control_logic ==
  state O2 [parallel]
    state A
      du:
      es_o.ego = es_i.ego;
      state O2_warmup
      state O2_normal
      state O2_failure
      (default) -> O2_warmup
      O2_warmup -> O2_normal : [after(480,tick)]
      O2_failure -> O2_normal : [es_i.ego < max_ego] / Fail.DEC;
      O2_normal -> O2_failure : [es_i.ego > max_ego] / Fail.INC;
    (default) -> A
  state Pressure [parallel]
    state normal
      du:
      es_o.map = es_i.map;
    state fail
      du:
      es_o.map = map_estimate(es_i.speed, es_i.throttle);
    state map = map_estimate(speed, throttle) [function]
    (default) -> normal
    fail -> normal : [es_i.map > min_press & ... es_i.map < max_press] / Fail.DEC;
    normal -> fail : [es_i.map > max_press | ... es_i.map < min_press] / Fail.INC;
  state Throttle [parallel]
    state normal
      du:
      es_o.throttle = es_i.throttle;
    state fail
      du:
      es_o.throttle = throttle_estimate(es_i.speed,es_i.map);
    state throttle = throttle_estimate(speed, map) [function]
    (default) -> normal
    fail -> normal : [es_i.throttle >  min_throt & ... es_i.throttle < max_throt] / Fail.DEC;
    normal -> fail : [es_i.throttle> max_throt | ... es_i.throttle < min_throt] / Fail.INC;
  state Speed [parallel]
    state normal
      du:
      es_o.speed = es_i.speed;
    state fail
      du:
      es_o.speed = speed_estimate(es_i.throttle, es_i.map);
    state speed = speed_estimate(throttle, map) [function]
    (default) -> normal
    fail -> normal : [es_i.speed > 0C] / Fail.DEC;
    normal -> fail : [es_i.speed == 0C & ... es_i.map < zero_thresh] / Fail.INC;
  state Fail [parallel]
    state Multi
      state Three
      state Four
      state Two
      Three -> Four : INC
      Two -> Three : INC
      Four -> Three : DEC
      Three -> Two : DEC
    state One
    state None
    (default) -> None
    One -> Two : INC
    Two -> One : DEC
    One -> None : DEC
  state Fueling_Mode [parallel]
    state Fuel_Disabled
      en:
      fuel_mode = DISABLED;
      state Overspeed
      state Shutdown
      Overspeed -> (junction 67) : [in(Speed.normal) & ... es_i.speed < (max_speed - hys)]
      (junction 67) -> Shutdown : [in(Fail.Multi)]
    state Running
      state Low_Emissions
        en:
        fuel_mode = LOW;
        state Warmup
        state Normal
        Warmup -> (junction 68) : [in(O2.A.O2_normal)]
        (junction 68) -> Normal
      state Rich_Mixture
        en:
        fuel_mode = RICH;
        state Single_Failure
      (junction 68) -> Single_Failure : [in(Fail.One)]
      Normal -> Single_Failure : [in(Fail.One)]
      Single_Failure -> Normal : [in(Fail.None)]
    (default) -> Warmup : {es_o = es_i;}
    Running -> Overspeed : [es_i.speed > max_speed]
    (junction 67) -> Running : [!in(Fail.Multi)]
    Running -> Shutdown : enter(Fail.Multi)
    Shutdown -> Rich_Mixture : exit(Fail.Multi)
  data: speed function_input s16En3; throttle function_input s16En3; map function_output; speed function_input s16En3; map function_input u8En7; throttle function_output; throttle function_input s16En3; map function_input u8En7; speed function_output; es_o output EngSensors; O2_normal output boolean; max_ego parameter s16En7 [0..2]; max_press parameter u8En7 [0..2]; min_press parameter u8En7 [0..2]; min_throt parameter s16En3 [0..120]; max_throt parameter s16En3 [0..120]; zero_thresh parameter u8En7 [0..450]; max_speed parameter s16En3 [0..1000]; hys parameter s16En3 [0..1000]; es_i input EngSensors; fuel_mode output Enum: sld_FuelModes [1..3] =sld_FuelModes.LOW
  events: local EITHER_EDGE_EVENT; local EITHER_EDGE_EVENT

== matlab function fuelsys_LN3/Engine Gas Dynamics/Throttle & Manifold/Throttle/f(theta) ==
function y = f(u)
%#codegen

y = 2.821 - 0.05231*u + 0.10299*u^2 - 0.00063*u^3;

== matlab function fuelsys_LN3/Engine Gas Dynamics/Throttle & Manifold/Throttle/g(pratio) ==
function y = g(u)
%#codegen

y = 2*sqrt(u - u^2);

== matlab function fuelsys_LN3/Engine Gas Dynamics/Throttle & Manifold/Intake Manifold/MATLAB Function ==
function y = pumping(u1,u2)
%#codegen

y = -0.366 + 0.08979*u1*u2 - 0.0337*u2*u1^2 + 0.0001*u1*u2^2;

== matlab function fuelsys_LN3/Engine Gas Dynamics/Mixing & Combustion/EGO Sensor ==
function y = fcn(u)
%#codegen

y = (1-tanh(4*(u-14.6)))/2;

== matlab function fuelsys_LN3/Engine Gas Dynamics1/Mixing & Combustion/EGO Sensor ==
function y = fcn(u)
%#codegen

y = (1-tanh(4*(u-14.6)))/2;

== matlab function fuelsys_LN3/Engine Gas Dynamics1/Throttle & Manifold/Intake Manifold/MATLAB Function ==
function y = pumping(u1,u2)
%#codegen

y = -0.366 + 0.08979*u1*u2 - 0.0337*u2*u1^2 + 0.0001*u1*u2^2;

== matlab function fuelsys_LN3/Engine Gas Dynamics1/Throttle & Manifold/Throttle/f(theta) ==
function y = f(u)
%#codegen

y = 2.821 - 0.05231*u + 0.10299*u^2 - 0.00063*u^3;

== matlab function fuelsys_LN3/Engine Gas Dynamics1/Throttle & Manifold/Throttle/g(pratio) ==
function y = g(u)
%#codegen

y = 2*sqrt(u - u^2);

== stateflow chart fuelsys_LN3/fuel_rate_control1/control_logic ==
  state O2 [parallel]
    state A
      du:
      es_o.ego = es_i.ego;
      state O2_warmup
      state O2_normal
      state O2_failure
      (default) -> O2_warmup
      O2_warmup -> O2_normal : [after(480,tick)]
      O2_failure -> O2_normal : [es_i.ego < max_ego] / Fail.DEC;
      O2_normal -> O2_failure : [es_i.ego > max_ego] / Fail.INC;
    (default) -> A
  state Pressure [parallel]
    state normal
      du:
      es_o.map = es_i.map;
    state fail
      du:
      es_o.map = map_estimate(es_i.speed, es_i.throttle);
    state map = map_estimate(speed, throttle) [function]
    (default) -> normal
    fail -> normal : [es_i.map > min_press & ... es_i.map < max_press] / Fail.DEC;
    normal -> fail : [es_i.map > max_press | ... es_i.map < min_press] / Fail.INC;
  state Throttle [parallel]
    state normal
      du:
      es_o.throttle = es_i.throttle;
    state fail
      du:
      es_o.throttle = throttle_estimate(es_i.speed,es_i.map);
    state throttle = throttle_estimate(speed, map) [function]
    (default) -> normal
    fail -> normal : [es_i.throttle >  min_throt & ... es_i.throttle < max_throt] / Fail.DEC;
    normal -> fail : [es_i.throttle> max_throt | ... es_i.throttle < min_throt] / Fail.INC;
  state Speed [parallel]
    state normal
      du:
      es_o.speed = es_i.speed;
    state fail
      du:
      es_o.speed = speed_estimate(es_i.throttle, es_i.map);
    state speed = speed_estimate(throttle, map) [function]
    (default) -> normal
    fail -> normal : [es_i.speed > 0C] / Fail.DEC;
    normal -> fail : [es_i.speed == 0C & ... es_i.map < zero_thresh] / Fail.INC;
  state Fail [parallel]
    state Multi
      state Three
      state Four
      state Two
      Three -> Four : INC
      Two -> Three : INC
      Four -> Three : DEC
      Three -> Two : DEC
    state One
    state None
    (default) -> One
    None -> One : INC
    Two -> One : DEC
  state Fueling_Mode [parallel]
    state Fuel_Disabled
      en:
      fuel_mode = DISABLED;
      state Overspeed
      state Shutdown
      Overspeed -> (junction 67) : [in(Speed.normal) & ... es_i.speed < (max_speed - hys)]
      (junction 67) -> Shutdown : [in(Fail.Multi)]
    state Running
      state Low_Emissions
        en:
        fuel_mode = LOW;
        state Warmup
        state Normal
        Warmup -> (junction 68) : [in(O2.A.O2_normal)]
        (junction 68) -> Normal
      state Rich_Mixture
        en:
        fuel_mode = RICH;
        state Single_Failure
      (junction 68) -> Single_Failure : [in(Fail.One)]
      Normal -> Single_Failure : [in(Fail.One)]
      Single_Failure -> Normal : [in(Fail.None)]
    (default) -> Warmup : {es_o = es_i;}
    Running -> Overspeed : [es_i.speed > max_speed]
    (junction 67) -> Running : [!in(Fail.Multi)]
    Running -> Shutdown : enter(Fail.Multi)
    Shutdown -> Rich_Mixture : exit(Fail.Multi)
  data: speed function_input s16En3; throttle function_input s16En3; map function_output; speed function_input s16En3; map function_input u8En7; throttle function_output; throttle function_input s16En3; map function_input u8En7; speed function_output; es_o output EngSensors; O2_normal output boolean; max_ego parameter s16En7 [0..2]; max_press parameter u8En7 [0..2]; min_press parameter u8En7 [0..2]; min_throt parameter s16En3 [0..120]; max_throt parameter s16En3 [0..120]; zero_thresh parameter u8En7 [0..450]; max_speed parameter s16En3 [0..1000]; hys parameter s16En3 [0..1000]; es_i input EngSensors; fuel_mode output Enum: sld_FuelModes [1..3] =sld_FuelModes.LOW
  events: local EITHER_EDGE_EVENT; local EITHER_EDGE_EVENT
